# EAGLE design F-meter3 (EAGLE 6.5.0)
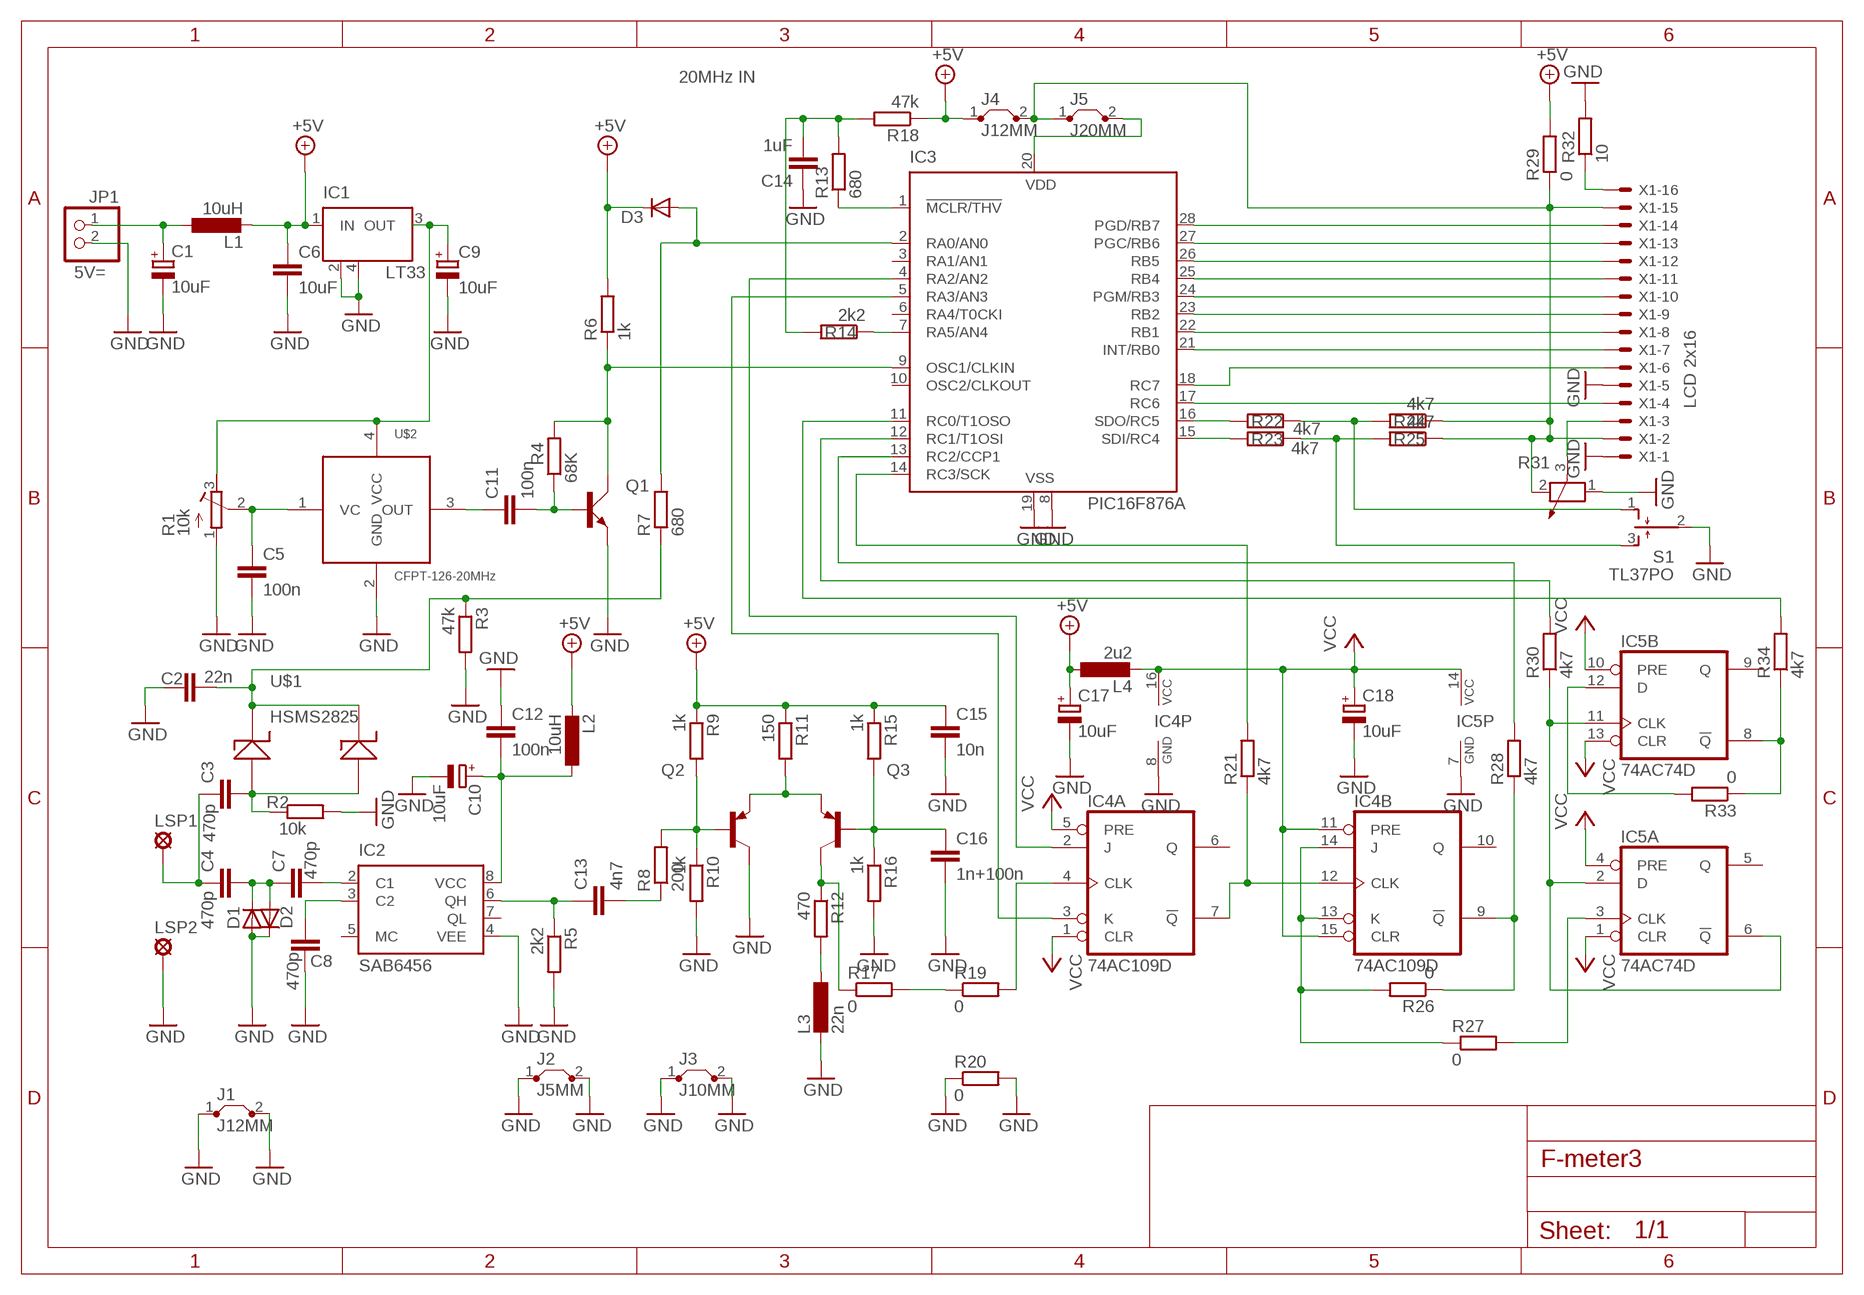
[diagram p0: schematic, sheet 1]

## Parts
C1  10uF  CPOL-EUE5-10.5  [E5-10,5]
C2  22n  C-EUC1206  [C1206]
C3  470p  C-EUC1206  [C1206]
C4  470p  C-EUC1206  [C1206]
C5  100n  C-EUC1206  [C1206]
C6  10uF  C-EUC1206  [C1206]
C7  470p  C-EUC1206  [C1206]
C8  470p  C-EUC1206  [C1206]
C9  10uF  CPOL-EU085CS-1AW  [085CS_1AW]
C10  10uF  CPOL-EUCT6032  [CT6032]
C11  100n  C-EUC1206  [C1206]
C12  100n  C-EUC1206  [C1206]
C13  4n7  C-EUC1206  [C1206]
C14  1uF  C-EUC1206  [C1206]
C15  10n  C-EUC1206  [C1206]
C16  1n+100n  C-EUC1206  [C1206]
C17  10uF  CPOL-EUCT6032  [CT6032]
C18  10uF  CPOL-EUCT6032  [CT6032]
D1  DIODE-MINIMELF  [MINIMELF]
D2  DIODE-MINIMELF  [MINIMELF]
D3  DIODE-MELF-MLL41  [MELF-MLL41]
IC1  LT33  LM340S  [SOT223]
IC2  SAB6456  [DIL08]
IC3  PIC16F876A  PIC16F876SO  [SO28W]
IC4  74AC109D  [SO16]
IC5  74AC74D  [SO14]
J1  J12MM  [12]
J2  J5MM  [05]
J3  J10MM  [10]
J4  J12MM  [12]
J5  J20MM  [20]
JP1  PINHD-1X02_2.54  [1X02]
L1  10uH  L-EUIRF-24  [IRF24]
L2  10uH  L-EUL1812  [L1812]
L3  22n  L-EUL1812  [L1812]
L4  2u2  L-EUL1812  [L1812]
LSP1  MCS10B  [MCS10B]
LSP2  MCS10B  [MCS10B]
Q1  BC847  2SC3838T146  [SC59]
Q2  BC808-25SMD  [SOT23-BEC]
Q3  BC808-25SMD  [SOT23-BEC]
R1  10k  R-TRIMM64X  [RTRIM64X]
R2  10k  R-EU_M1206  [M1206]
R3  47k  R-EU_M1206  [M1206]
R4  68K  R-EU_M1206  [M1206]
R5  2k2  R-EU_M1206  [M1206]
R6  1k  R-EU_M1206  [M1206]
R7  680  R-EU_M1206  [M1206]
R8  200  R-EU_M1206  [M1206]
R9  1k  R-EU_M1206  [M1206]
R10  1k  R-EU_M1206  [M1206]
R11  150  R-EU_M1206  [M1206]
R12  470  R-EU_M1206  [M1206]
R13  680  R-EU_M1206  [M1206]
R14  2k2  R-EU_M1206  [M1206]
R15  1k  R-EU_M1206  [M1206]
R16  1k  R-EU_M1206  [M1206]
R17  0  R-EU_M1206  [M1206]
R18  47k  R-EU_M1206  [M1206]
R19  0  R-EU_M1206  [M1206]
R20  0  R-EU_M1206  [M1206]
R21  4k7  R-EU_M1206  [M1206]
R22  4k7  R-EU_M1206  [M1206]
R23  4k7  R-EU_M1206  [M1206]
R24  4k7  R-EU_M1206  [M1206]
R25  4k7  R-EU_M1206  [M1206]
R26  0  R-EU_M1206  [M1206]
R27  0  R-EU_M1206  [M1206]
R28  4k7  R-EU_M1206  [M1206]
R29  0  R-EU_M1206  [M1206]
R30  4k7  R-EU_M1206  [M1206]
R31  POTENTIOMETER_PT-10S  [PT-10S]
R32  10  R-EU_M1206  [M1206]
R33  0  R-EU_M1206  [M1206]
R34  4k7  R-EU_M1206  [M1206]
S1  TL37PO  [TL3XPO]
U$1  HSMS2825  [HSMS2825]
U$2  CFPT-126-20MHz  CFPT-126  [CFPT-126]
X1  LCD 2x16  C-GRID-16-70543  [70543-16]

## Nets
GND: C1.- C2.1 C5.2 C6.2 C8.1 C9.- C10.- C12.1 C14.1 C15.2 C16.2 C17.- C18.- D1.A D2.C IC1.2(GND) IC1.4(GND) IC2.4(VEE) IC3.8(VSS) IC3.19(VSS) IC4.8(P:GND) IC5.7(P:GND) J1.1 J1.2 J2.1 J2.2 J3.1 J3.2 JP1.2 L3.2 LSP2.MP Q1.E Q2.C R1.1(A) R2.2 R3.2 R5.2 R10.2 R16.2 R20.1 R20.2 R31.1 R32.2 S1.2(P) U$2.2(GND) X1.1 X1.5
N$2: IC3.20(VDD) J5.2
N$3: J4.2 J5.1 R24.1 R25.1 R29.1 R31.2 X1.2 X1.15
N$6: C6.1 C15.1 C17.+ D3.C IC1.1(IN) J4.1 L1.2 L2.2 L4.1 R6.2 R9.1 R11.1 R15.1 R18.1 R29.2 ; supply symbol labelled +5V
N$11: IC3.17(RC6) X1.4
N$12: IC3.18(RC7) X1.6
N$13: IC3.21(INT/RB0) X1.7
N$14: C2.2 R3.1 R7.1 U$1.P$1(K2) U$1.P$2(K1)
N$15: IC3.23(RB2) X1.9
N$16: IC3.24(PGM/RB3) X1.10
N$17: IC3.25(RB4) X1.11
N$18: IC3.26(RB5) X1.12
N$19: IC3.27(PGC/RB6) X1.13
N$20: IC3.28(PGD/RB7) X1.14
N$21: C14.2 R13.2 R14.2 R18.2
N$23: C3.2 R2.1 U$1.P$3(A1) U$1.P$4(A2)
N$24: R32.1 X1.16
N$25: C11.1 U$2.3(OUT)
N$26: C11.2 Q1.B R4.1
N$27: IC3.9(OSC1/CLKIN) Q1.C R4.2 R6.1
N$28: R31.3 X1.3
N$29: IC4.13(B:K) IC4.14(B:J) R26.2 R27.1
N$30: Q2.B R8.2 R9.2 R10.1
N$31: IC5.8(B:!Q) R33.1 R34.1
N$32: C16.1 Q3.B R15.2 R16.1
N$33: L3.1 R12.2
N$34: Q2.E Q3.E R11.2
N$35: IC4.4(A:CLK) R19.2
N$36: IC3.4(RA2/AN2) IC4.2(A:J)
N$37: IC3.5(RA3/AN3) IC4.3(A:K)
N$38: IC3.7(RA5/AN4) R14.1
N$40: IC4.9(B:!Q) R26.1 R28.1
N$42: IC4.7(A:!Q) IC4.12(B:CLK) R21.1
N$44: IC3.11(RC0/T1OSO) R34.2
N$45: IC3.12(RC1/T1OSI) R30.2
N$46: IC3.13(RC2/CCP1) R28.2
N$47: IC3.14(RC3/SCK) R21.2
N$48: C7.2 IC2.2(C1)
N$49: IC3.22(RB1) X1.8
N$50: C13.2 R8.1
N$51: C13.1 IC2.6(QH) R5.1
N$52: C9.+ IC1.3(OUT) R1.3(E) U$2.4(VCC)
N$53: C5.1 R1.2(S) U$2.1(VC)
N$56: IC3.16(SDO/RC5) R22.2
N$57: C4.2 C7.1 D1.C D2.A
N$58: C3.1 C4.1 LSP1.MP
N$59: C10.+ C12.2 IC2.8(VCC) L2.1
N$60: C8.2 IC2.3(C2)
N$63: IC3.15(SDI/RC4) R23.2
N$64: R22.1 R24.2 S1.1(O)
N$65: R23.1 R25.2 S1.3(S)
N$66: IC5.12(B:D) R33.2
N$67: IC5.2(A:D) IC5.6(A:!Q) IC5.11(B:CLK) R30.1
N$68: IC5.3(A:CLK) R27.2
N$69: R17.2 R19.1
N$70: Q3.C R12.1 R17.1
N$73: D3.A IC3.2(RA0/AN0) R7.2
N$78: C1.+ JP1.1 L1.1
N$79: IC3.1(!MCLR/THV) R13.1
VCC: C18.+ IC4.1(A:CLR) IC4.5(A:PRE) IC4.11(B:PRE) IC4.15(B:CLR) IC4.16(P:VCC) IC5.1(A:CLR) IC5.4(A:PRE) IC5.10(B:PRE) IC5.13(B:CLR) IC5.14(P:VCC) L4.2
Unconnected: IC2.5(MC) IC2.7(QL) IC3.3(RA1/AN1) IC3.6(RA4/T0CKI) IC3.10(OSC2/CLKOUT) IC4.6(A:Q) IC4.10(B:Q) IC5.5(A:Q) IC5.9(B:Q)

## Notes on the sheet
- 20MHz IN
- 5V=

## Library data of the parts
C1 C10 C17 C18 = rcl:CPOL-EU: POLARIZED CAPACITOR, European symbol
C2-C8 C11-C16 = rcl:C-EU: CAPACITOR, European symbol
C9 = rcl-2:CPOL-EU: POLARIZED CAPACITOR, European symbol
D1-D3 = diode-1:DIODE-: DIODE
IC1 = linear:LM340S: 3-Terminal Positive Regulators Source: http://cache.national.com/ds/LM/LM340.pdf
IC2 = philips-semiconductors:SAB6456: Sensitive 1 GHz divide-by-64/divide-by-256 switchable prescaler Source: PHILIPS .. SAB6456.pdf; OC_FARNELL: unknown; OC_NEWARK: unknown
IC3 = microchip:PIC16*876: MICROCONTROLLER flash type; MF: MICROCHIP; MPN: PIC16F876-20/SO; OC_FARNELL: 9761268; OC_NEWARK: 12C1950
IC4 = 74xx-eu:74*109: Dual J-K positive edge triggered FLIP FLOP, preset and clear
IC5 = 74xx-eu:74*74: Dual D type positive edge triggered FLIP FLOP, preset and clear
J1-J5 = jumper:J: Bridge
JP1 = pinhead-2:PINHD-1X02: PIN HEADER
L1-L4 = rcl:L-EU: INDUCTOR, European symbol
LSP1 LSP2 = solpad:MCS10B: SOLDER PAD
Q1 = transistor-small-signal:2SC3838: High-Frequency Amplifier Transistor 11V, 50mA, 3.2GHz (Rohm)
Q2 Q3 = transistor-pnp:BC808*: PNP Transistror
R1 = rcl:R-TRIMM: Trimm resistor
R2-R30 R32-R34 = rcl:R-EU_: RESISTOR, European symbol
R31 = rcl:POTENTIOMETER_: Potentiometer
S1 = switch:TL37PO: TINY SWITCH MOM OFF MOM Source: http://www2.produktinfo.conrad.com/datenblaetter/700000-724999/705152-da-01-de-Subminiaturschalter_TL_36YO.pdf
U$1 = HSMS2825:HSMS2825
U$2 = CFPT-126:CFPT-126: Generator TCVCXO typ CFPT-126
X1 = con-molex:C-GRID-16: CONNECTOR wire to board 2.54 mm (0.100") pitch header; OC_FARNELL: unknown; OC_NEWARK: unknown

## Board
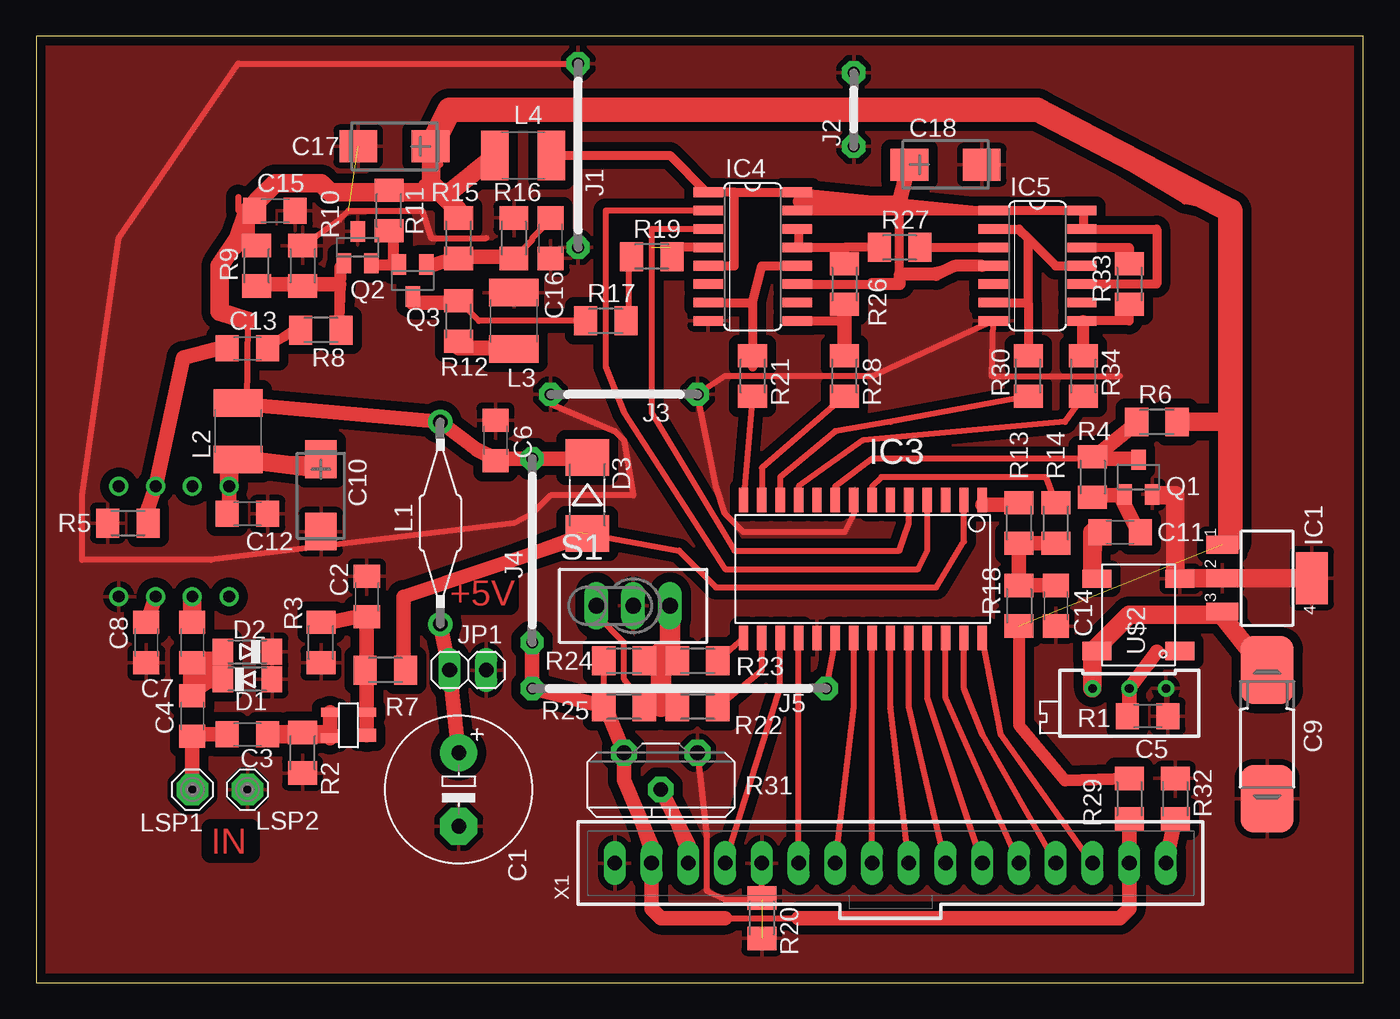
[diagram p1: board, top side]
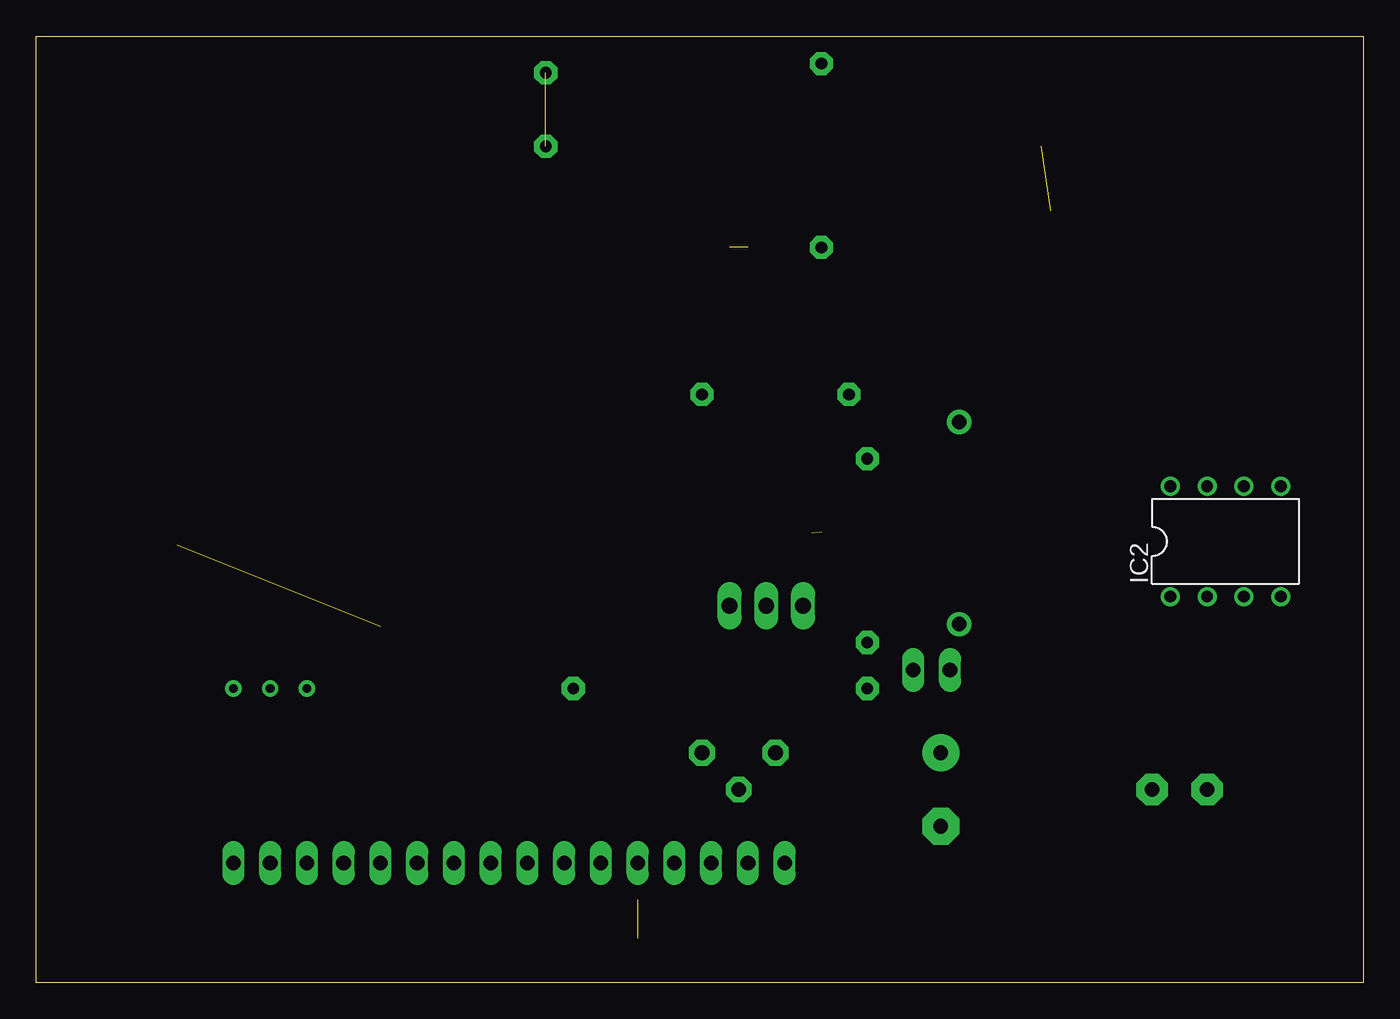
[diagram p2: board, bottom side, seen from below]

Size 91.75 x 65.39 mm. Coordinates in mm from the lower left corner, seen from the top.
Outline: 0,0 91.75,0 91.75,65.39 0,65.39 0,0
Copper layers (1*16): Top 0.035mm / dielectric 1.5mm / Bottom 0.035mm
Design rules "default *": minimum track width 16mil, minimum drill 24mil, track to track 8mil, track to pad 8mil, pad to pad 8mil, via to via 8mil, smd to smd 8mil, copper to edge 10mil, drill to drill 8mil, minimum pad ring 10mil, minimum via ring 8mil, stop-mask expansion 4mil, vias tented up to drill 0mil, thermal gap 16mil

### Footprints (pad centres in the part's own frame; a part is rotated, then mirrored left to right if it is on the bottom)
E5-10,5 = drill 1.016 pad 2.54: + -2.54,0 | drill 1.016 pad 2.54 octagon: - 2.54,0
C1206 = smd 1.6 x 1.8: 1 -1.4,0; 2 1.4,0
085CS_1AW = smd 4.7 x 3.7: + 4.45,0; - -4.45,0
CT6032 = smd 2.6 x 2.2: + -2.5,0; - 2.5,0
MINIMELF = smd 1.4 x 1.8: A 1.7,0; C -1.7,0
MELF-MLL41 = smd 2.5 x 3: A 2.625,0; C -2.625,0
SOT223 = smd 1.219 x 2.235: 1 -2.311,-3.099; 2 0,-3.099; 3 2.311,-3.099 | smd 3.6 x 2.2: 4 0,3.099
DIL08 = drill 0.813 pad 1.27: 1 -3.81,-3.81; 2 -1.27,-3.81; 3 1.27,-3.81; 4 3.81,-3.81; 5 3.81,3.81; 6 1.27,3.81; 7 -1.27,3.81; 8 -3.81,3.81
SO28W = smd 0.65 x 1.7: 1 -7.62,-4.78; 2 -6.35,-4.78; 3 -5.08,-4.78; 4 -3.81,-4.78; 5 -2.54,-4.78; 6 -1.27,-4.78; 7 0,-4.78; 8 1.27,-4.78; 9 2.54,-4.78; 10 3.81,-4.78; 11 5.08,-4.78; 12 6.35,-4.78; 13 7.62,-4.78; 14 8.89,-4.78; 15 8.89,4.78; 16 7.62,4.78; 17 6.35,4.78; 18 5.08,4.78; 19 3.81,4.78; 20 2.54,4.78; 21 1.27,4.78; 22 0,4.78; 23 -1.27,4.78; 24 -2.54,4.78; 25 -3.81,4.78; 26 -5.08,4.78; 27 -6.35,4.78; 28 -7.62,4.78
SO16 = smd 0.66 x 2.032: 1 -4.445,-3.073; 2 -3.175,-3.073; 3 -1.905,-3.073; 4 -0.635,-3.073; 5 0.635,-3.073; 6 1.905,-3.073; 7 3.175,-3.073; 8 4.445,-3.073; 9 4.445,3.073; 10 3.175,3.073; 11 1.905,3.073; 12 0.635,3.073; 13 -0.635,3.073; 14 -1.905,3.073; 15 -3.175,3.073; 16 -4.445,3.073
SO14 = smd 0.66 x 2.032: 1 -3.81,-3.073; 2 -2.54,-3.073; 3 -1.27,-3.073; 4 0,-3.073; 5 1.27,-3.073; 6 2.54,-3.073; 7 3.81,-3.073; 8 3.81,3.073; 9 2.54,3.073; 10 1.27,3.073; 11 0,3.073; 12 -1.27,3.073; 13 -2.54,3.073; 14 -3.81,3.073
12 = drill 0.813 pad 1.6 octagon: 1 -6.35,0; 2 6.35,0
05 = drill 0.813 pad 1.6 octagon: 1 -2.54,0; 2 2.54,0
10 = drill 0.813 pad 1.6 octagon: 1 -5.08,0; 2 5.08,0
20 = drill 0.813 pad 1.6 octagon: 1 -10.16,0; 2 10.16,0
1X02 = drill 1.016 long: 1 -1.27,0; 2 1.27,0
IRF24 = drill 1 pad 1.676: 1 -6.985,0; 2 6.985,0
L1812 = smd 1.9 x 3.4: 1 -1.95,0; 2 1.95,0
MCS10B = drill 1.016 pad 2.159 octagon: MP 0,0
SC59 = smd 1 x 1.4: B -0.95,-1.2; C 0,1.2; E 0.95,-1.2
SOT23-BEC = smd 1 x 1.4: B -0.95,-1.1; C 0,1.1; E 0.95,-1.1
RTRIM64X = drill 0.61: 1 1.27,-2.54; 2 1.27,0; 3 1.27,2.54
M1206 = smd 1.6 x 2: 1 -1.4,0; 2 1.4,0
PT-10S = drill 1.016 pad 1.778 octagon: 1 -2.54,-1.27; 2 2.54,-1.27; 3 0,1.27
TL3XPO = drill 1.1 pad 1.422 long: 1 -2.54,0; 2 0,0; 3 2.54,0
HSMS2825 = smd 0.914 x 1.27: P$1 -0.699,-1.27 | smd 0.635 x 1.27: P$2 0.889,-1.27; P$3 0.889,1.27; P$4 -0.889,1.27
CFPT-126 = smd 1.27 x 2: 1 -2.5,-2.862; 2 2.5,-2.862; 3 2.5,2.862; 4 -2.5,2.862
70543-16 = drill 1.016 long: 1 -19.05,0; 2 -16.51,0; 3 -13.97,0; 4 -11.43,0; 5 -8.89,0; 6 -6.35,0; 7 -3.81,0; 8 -1.27,0; 9 1.27,0; 10 3.81,0; 11 6.35,0; 12 8.89,0; 13 11.43,0; 14 13.97,0; 15 16.51,0; 16 19.05,0

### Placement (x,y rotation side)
C1  29.21,13.34 270 top
C2  22.86,26.67 270 top
C3  14.61,17.14 0 top
C4  10.79,18.41 90 top
C5  76.83,18.41 0 top
C6  31.75,37.47 90 top
C7  10.79,23.5 90 top
C8  7.62,23.5 90 top
C9  85.09,17.14 90 top
C10  19.68,33.66 270 top
C11  74.93,31.11 0 top
C12  14.61,32.38 180 top
C13  14.61,43.81 0 top
C14  70.48,26.04 90 top
C15  16.51,53.34 0 top
C16  35.56,51.44 270 top
C17  24.77,57.78 180 top
C18  62.87,56.52 0 top
D1  14.61,20.95 0 top
D2  14.61,22.86 180 top
D3  38.1,33.66 270 top
IC1  85.09,27.94 270 top
IC2  9.53,30.48 0 bottom
IC3  57.78,28.57 180 top
IC4  49.53,50.16 270 top
IC5  69.22,49.53 270 top
J1  37.47,57.15 90 top
J2  56.52,60.33 90 top
J3  40.64,40.64 180 top
J4  34.29,29.84 270 top
J5  44.45,20.32 0 top
JP1  29.84,21.59 0 top
L1  27.94,31.75 90 top
L2  13.97,38.1 90 top
L3  33.02,45.72 90 top
L4  33.66,57.15 0 top
LSP1  10.79,13.34 90 top
LSP2  14.61,13.34 90 top
Q1  76.2,34.92 0 top
Q2  22.23,50.8 0 top
Q3  26.04,48.51 180 top
R1  75.56,19.05 90 top
R2  18.41,15.88 270 top
R3  19.68,23.5 270 top
R4  73.03,34.92 90 top
R5  6.35,31.75 180 top
R6  77.47,38.73 0 top
R7  24.13,21.59 0 top
R8  19.68,45.09 0 top
R9  15.24,49.53 270 top
R10  18.41,49.53 90 top
R11  24.38,53.34 270 top
R12  29.21,45.72 270 top
R13  67.94,31.75 270 top
R14  70.48,31.75 270 top
R15  29.21,51.44 270 top
R16  33.02,51.44 90 top
R17  39.37,45.72 0 top
R18  67.94,26.04 90 top
R19  42.55,50.16 0 top
R20  50.16,4.45 90 top
R21  49.53,41.91 270 top
R22  45.72,19.05 0 top
R23  45.72,22.23 0 top
R24  40.64,19.05 0 top
R25  40.64,22.23 0 top
R26  55.88,48.26 90 top
R27  59.69,50.8 0 top
R28  55.88,41.91 270 top
R29  75.56,12.7 90 top
R30  68.58,41.91 270 top
R31  43.18,14.61 180 top
R32  78.74,12.7 90 top
R33  75.56,48.26 90 top
R34  72.39,41.91 270 top
S1  41.27,26.04 0 top
U$1  21.59,17.78 90 top
U$2  76.2,25.4 90 top
X1  59.05,8.26 0 top

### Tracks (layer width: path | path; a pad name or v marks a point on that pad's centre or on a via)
GND  (3 unrouted)
  Top 0.406: R10.2 20.95,52.7 21.59,53.34 26.67,53.34 27.3,51.44 31.11,51.44 | 45.72,16.19 R31.1 46.35,10.16 46.35,6.35 47.62,5.71 50.16,5.71 X1.5 | IC3.8 56.52,32.38 55.88,31.11 48.9,31.11 47.62,32.38 46.99,34.29 J3.1 | U$2.2 78.74,33.66 | 77.47,33.66 76.83,33.66 | 74.93,41.91 66.04,41.91 IC5.7 57.78,41.91 47.62,41.91 J3.1 | L3.2 33.66,47.62 | J3.2 35.56,40.01 40.01,38.1 40.64,37.47 41.27,33.66 35.56,33.66 34.29,32.38 33.02,31.75 12.06,29.21 3.17,29.21 3.17,33.66 5.71,51.44 13.97,63.5 J1.2 | 45.09,40.64 J3.1 | 70.48,24.77 C14.1 70.48,24.13
  Top 1.27: 77.47,33.66 78.74,33.66 78.74,27.94 88.27,27.94
  pour Top (isolate 0.635): 0,92.71 117.47,92.71 117.47,0 0,0
N$1
  Top 1.27: 73.03,27.94 73.03,31.11
N$2
  Top 0.406: IC3.20 J5.2
N$3
  Top 0.406: 47.62,4.45 52.7,4.45 | 75.56,5.08 X1.15 75.56,10.79 R29.1 | R24.1 R25.1 | X1.2 40.64,13.97 | R31.2 R24.1 | R24.1 38.73,19.05 J5.1
  Top 1.016: J4.2 J5.1 39.37,19.05 R31.2 40.64,13.97 42.55,9.53 X1.2 42.55,5.08 43.18,4.45 47.62,4.45 | 75.56,10.79 75.56,5.08 74.93,4.45 52.7,4.45
N$5
  Top 1.016: 65.41,33.02 67.94,33.02
N$6  (1 unrouted)
  Top 0.406: 14.61,51.12 14.92,51.44 14.92,53.34 C15.1 15.24,53.34 16.83,54.93 24.13,54.93 R11.1 25.72,54.93 27.62,54.93 26.67,55.24 | 14.61,51.12 R9.1 | 26.67,55.24 27.94,56.52 C17.+ 28.57,59.69 69.85,59.69 79.38,53.98 82.55,53.34 82.55,38.73 IC1.1 | 28.26,53.98 26.99,55.24 26.67,55.24 | 28.26,53.98 29.21,53.02 R15.1 | 28.26,53.98 31.43,57.15 L4.1 | 12.7,49.53 14.61,51.12 | L2.2 14.54,40 | 14.54,40 L1.2 C6.1 D3.C J4.1 | 79.06,38.73 R6.2 78.74,38.73 | 13.97,54.29 13.97,53.34 14.54,53.15 | 14.61,45.72 14.54,40
  Top 0.813: R18.1 67.94,17.78 71.12,13.97 R29.2
  Top 1.016: 38.1,36.2 31.75,36.2 30.48,36.83 L1.2 13.97,40.01
  Top 1.27: 14.61,53.34 14.54,53.15 13.97,51.44 12.7,49.53 12.7,46.35 14.61,45.72 | R6.2 82.55,38.73
N$7
  Top 1.016: 73.03,33.66 74.93,33.66 76.2,31.11
N$11
  Top 0.406: X1.4 51.44,20.32 IC3.17
N$12
  Top 0.406: X1.6 IC3.18
N$13
  Top 0.406: X1.7 56.52,19.05 IC3.21
N$14
  Top 0.406: U$1.P$2 22.86,19.05 22.86,21.59 | 22.86,21.59 22.86,22.23 | 22.86,22.23 R7.1 22.86,21.59 | 22.86,22.23 C2.2 R3.1
  Top 1.016: 22.86,19.05 22.86,25.4 19.68,24.77 | U$1.P$2 U$1.P$1
N$15
  Top 0.406: X1.9 59.05,19.05 IC3.23
N$16
  Top 0.406: X1.10 60.33,19.05 IC3.24
N$17
  Top 0.406: X1.11 61.59,19.68 IC3.25
N$18
  Top 0.406: X1.12 62.87,19.68 IC3.26
N$19
  Top 0.406: X1.13 65.41,17.14 64.14,20.32 IC3.27
N$20
  Top 0.406: X1.14 66.67,17.14 IC3.28
N$21
  Top 1.016: C14.2 R18.2 R13.2 R14.2
N$23
  Top 0.406: R2.1 20.32,17.27 U$1.P$4
  Top 1.016: U$1.P$3 20.32,17.14 U$1.P$4
  Top 1.27: C3.2 20.32,17.14
N$24
  Top 0.406: X1.16 R32.1
  Top 1.016: X1.16 78.74,11.43
N$25
  Top 0.406: C11.1 U$2.3
N$26
  Top 0.406: R4.1 Q1.B C11.2
N$27
  Top 0.406: Q1.C R4.2 R6.1 73.03,36.2 57.78,36.2 55.24,34.29 IC3.9
  Top 1.016: 76.2,38.73 73.03,36.2 75.56,36.2
N$28
  Top 0.406: X1.3 R31.3
  Top 1.016: R31.3 45.09,9.53 X1.3
N$29
  Top 0.254: IC4.14 IC4.13 52.7,50.8 | R26.2 55.88,50.8 R27.1
  Top 0.61: 52.7,52.07 52.7,50.8 55.88,50.8 | 58.42,50.8 55.88,50.8 | 55.88,50.8 55.88,49.53
N$30
  Top 0.254: 20.95,49.53 21.27,49.53 Q2.B | 15.88,48.26 14.61,48.26 R9.2 | 18.41,48.26 R10.1
  Top 0.406: R8.2 Q2.B | R10.1 18.73,48.26 19.05,48.26
  Top 0.61: 20.95,45.09 20.95,48.26 20.95,49.53
  Top 1.016: 18.41,48.26 15.88,48.26 | 19.05,48.26 20.95,48.26
N$31
  Top 0.254: R33.1 75.56,46.35 | 73.03,45.72 72.39,45.72 IC5.8
  Top 0.406: 75.56,45.72 72.39,45.72
  Top 0.61: 75.56,46.35 75.56,45.72 73.03,45.72
  Top 0.813: 72.39,43.18 R34.1 72.39,45.72
N$32
  Top 0.254: Q3.B 26.99,49.85 29.21,49.85 R15.2 29.21,50.16 | 33.02,50.16 R16.1
  Top 0.406: C16.1 35.56,52.7 34.29,51.44 34.29,51.3 R16.1
  Top 1.016: 27.3,49.53 29.21,50.16 33.02,50.16
N$33
  Top 0.406: R12.2 29.21,44.13 32.7,44.13 33.02,43.81 L3.1
N$34
  Top 0.254: 24.45,49.85 23.18,49.85 Q2.E | 24.45,49.85 25.08,49.85 Q3.E | 24.45,49.85 24.45,51.75 R11.2
N$35  (1 unrouted)
  Top 0.406: 42.55,50.8 42.55,50.67 | IC4.4 46.35,50.8 | 44.45,50.8 43.81,50.8 43.81,50.3 R19.2
  Top 0.61: 46.35,50.8 44.45,50.8
N$36
  Top 0.406: IC4.2 39.37,53.34 39.37,42.55 40.64,39.37 47.62,28.57 60.96,28.57 61.59,29.84 IC3.4
N$37
  Top 0.406: 60.33,33.66 IC3.5 60.33,31.75 59.69,29.84 48.26,29.84 42.55,39.37 42.55,52.07 IC4.3
N$38
  Top 0.406: R14.1 69.85,34.92 58.42,34.92 57.78,34.29 IC3.7
N$40
  Top 0.254: R28.1 55.88,43.81 | 55.88,46.35 R26.1 | IC4.9 52.7,45.72
  Top 0.61: 52.7,45.72 55.88,45.72
  Top 1.016: 55.88,46.99 55.88,46.35 55.88,45.72 55.88,43.81
N$41
  Top 1.27: 31.75,57.15 28.57,54.61 20.32,54.61 19.68,55.24 16.51,55.24 15.24,53.98
N$42
  Top 0.254: 52.7,49.53 IC4.12 51.44,49.53 | 47.62,46.99 49.53,46.99 R21.1
  Top 0.406: 47.62,46.99 46.99,46.99 IC4.7
  Top 0.61: 46.99,46.99 49.53,46.99 | 49.53,46.99 49.53,42.55 | 49.53,46.99 50.16,49.53 51.44,49.53
N$44
  Top 0.406: R34.2 71.12,38.73 57.15,37.47 52.7,34.29 IC3.11
N$45
  Top 0.406: R30.2 59.05,38.73 55.24,38.1 51.44,34.92 IC3.12
N$46
  Top 0.406: R28.2 50.16,35.56 IC3.13
N$47
  Top 0.406: R21.2 IC3.14
N$48
  Top 0.406: IC2.2 C7.2
  Top 1.27: IC2.2 10.79,24.77
N$49
  Top 0.406: X1.8 IC3.22
N$50
  Top 0.406: R8.1 C13.2
N$51
  Top 0.406: R5.1 IC2.6 | 10.16,43.18 C13.1
  Top 1.016: 7.62,32.38 IC2.6 10.16,43.18 12.7,43.81
N$52
  Top 0.406: R1.3 U$2.4 76.2,25.4 IC1.3 C9.+
  Top 1.27: R1.3 73.03,22.86 75.56,25.4 81.92,25.4 84.45,22.23
N$53
  Top 0.406: U$2.1 77.15,22.86 77.15,21.91 R1.2 C5.1
  Top 1.016: 77.47,22.86 R1.2 75.56,19.05
N$54
  Top 1.27: 19.05,35.56 13.97,36.2
N$56
  Top 0.406: R22.2 50.16,21.59 IC3.16
N$57
  Top 0.406: C4.2 10.79,20.95 C7.1 13.34,22.23 | 13.34,22.23 D1.C | 13.34,22.23 12.7,20.95 10.79,19.68 | D2.A 13.02,22.86 13.02,22.54 12.7,22.23
  Top 1.27: 10.79,19.68 10.79,20.95 | 10.79,20.95 10.79,22.23 12.7,22.23 12.7,20.95 10.79,20.95
N$58
  Top 0.406: LSP1.MP C4.1 C3.1
  Top 1.016: LSP1.MP 10.79,17.14 13.34,17.14
N$59
  Top 0.406: IC2.8 L2.1 C10.+ | C12.2 13.34,34.92
  Top 1.016: IC2.8 13.34,32.38
  Top 1.27: 13.34,35.56 13.34,34.92 IC2.8
N$60
  Top 0.406: IC2.3 C8.2
  Top 1.016: IC2.3 7.62,24.77
N$61
  Top 1.27: 27.3,57.78 27.3,55.24 29.21,53.34
  Top 1.676: 27.3,57.78 28.57,60.33 69.22,60.33 82.55,53.34 82.55,30.48
N$63
  Top 0.406: R23.2 IC3.15
N$64
  Top 0.406: R22.1 43.18,19.05 R24.2 40.64,20.95 40.64,23.5 38.73,25.4 S1.1
  Top 1.422: 43.18,19.05 43.18,22.86
N$65
  Top 0.406: R23.1 43.81,23.5 | 43.81,23.5 R25.2 | S1.3 43.81,23.5
  Top 1.422: S1.3 43.81,22.23
N$66
  Top 0.254: IC5.12 73.03,50.8 | 75.56,50.16 R33.2
  Top 0.61: 73.03,50.8 75.56,50.8 75.56,50.16
N$67
  Top 0.254: 66.04,52.07 IC5.2 66.67,52.07 | 71.75,49.53 IC5.11 | R30.1 68.58,46.99 | 66.67,46.99 IC5.6
  Top 0.61: 66.67,52.07 67.94,52.07 68.58,51.44 | 68.58,51.44 70.48,49.53 71.75,49.53 | 66.67,46.99 68.58,46.99 | 68.58,46.99 68.58,51.44 | 68.58,46.99 68.58,43.18
N$68
  Top 0.254: R27.2 66.04,50.8 IC5.3
  Top 0.61: 60.96,50.8 66.04,50.8
N$69
  Top 0.406: R17.2 40.96,45.72 40.96,50.16 R19.1
N$70
  Top 0.406: R17.1 30.61,45.72 R12.1 26.33,47.12 Q3.C
N$73  (1 unrouted)
  Top 0.406: 64.14,33.02 IC3.2 64.14,30.48 62.23,27.3 46.99,27.3 44.45,29.84 37.47,31.11 25.4,26.67 R7.2
  Top 1.016: 25.4,21.59 25.4,26.67 36.83,30.48
N$76
  Top 0.61: 15.88,43.81 17.78,45.09
N$77
  Top 0.61: 23.5,49.53 24.77,49.53 24.77,51.44
N$78
  Top 1.016: C1.+ JP1.1 L1.1
N$79
  Top 0.406: IC3.1 R13.1
N$82
  Top 1.016: 29.21,43.81 32.38,43.81
N$83
  Top 1.016: 26.04,46.99 29.21,46.99
VCC
  Top 0.254: IC5.14 72.39,53.34 73.03,53.34 | 48.26,54.61 IC4.16 59.69,53.95 59.75,53.94 | IC5.14 IC5.13 72.39,52.07 | IC5.14 71.75,53.34 | 66.67,53.34 IC5.1 59.75,53.94 | 73.03,48.26 IC5.10 | 46.99,49.53 IC4.5 | IC4.11 53.34,48.26 | 59.69,48.26 59.7,49.21 59.75,53.94
  Top 0.406: 46.99,54.61 IC4.1 46.35,54.61 | 52.7,54.61 IC4.16 | 52.7,53.34 IC4.15 | 65.41,49.53 IC5.4 | 63.5,49.53 61.91,49.21 59.69,49.21 59.7,49.21 | C18.+ 59.69,53.98 59.69,53.95 | 43.81,57.15 L4.2
  Top 0.61: 53.34,53.34 59.69,53.34 | 59.69,53.34 65.41,53.34 52.7,54.61 | 46.99,49.53 48.26,49.53 48.26,54.61 | 48.26,54.61 46.99,54.61 46.35,54.61 43.81,57.15 35.56,57.15 | 48.26,54.61 52.7,54.61 | 72.39,53.34 72.39,52.07 77.47,52.07 77.47,48.26 73.03,48.26 | 71.75,53.34 66.67,53.34 | 52.7,53.34 52.7,53.98 52.7,54.61 | 53.34,48.26 57.78,48.26 | 59.69,48.9 59.69,53.34
  Top 0.813: 65.41,49.53 63.5,49.53 62.23,48.9 59.69,48.9 59.69,48.26 57.78,48.26 | 52.7,53.98 59.69,53.98
  Top 1.016: 60.33,56.52 59.69,53.98

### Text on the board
Top: +5V | IN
